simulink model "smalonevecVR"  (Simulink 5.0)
settings: Solver=ode23t  StartTime=0.0  StopTime=4  MaxStep=0.01  RelTol=1e-5  AbsTol=1e-4
InitFcn:
  | smalonevecdef
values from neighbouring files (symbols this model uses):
  Ef = parEf(m)    [Ccurverun.m]
  Ra = .95    (= 0.95)    [altwdgs.m]    (also in Ccurverun.m = 0.018)
  wo = 2*pi*freq0    [calc0.m]    (also in IMabc2.m = 376.991118431; imabcparam.m = 376.991118431; IMabcrun0.m = 376.991118431; IMabcrun1.m = 376.991118431)
undefined symbols (not defined in the file or in its folder): fa0, fk0, L_1, phif0, Rf, Rkd, Rkq, vf0

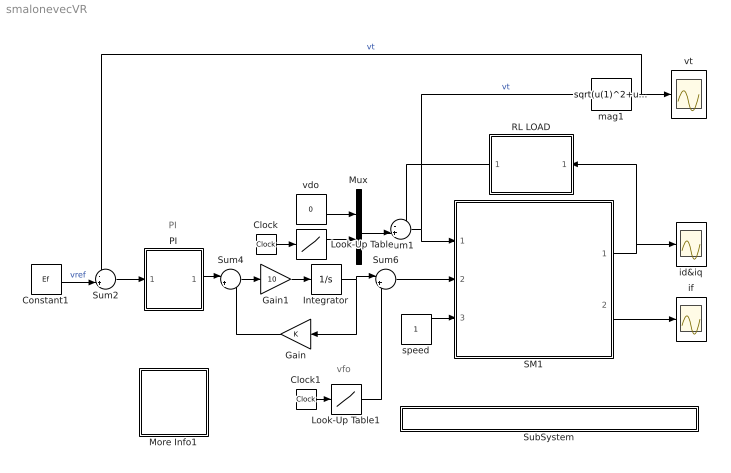
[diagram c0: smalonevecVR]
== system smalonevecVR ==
  note: vfo
  note: PI
  Clock : Clock
  Clock1 : Clock
  Constant1 : Constant  Value=Ef
  Gain : Gain  Orientation=left
  Gain1 : Gain  Gain=10
  Integrator : Integrator
  Look-Up Table : Lookup  InputValues=[0 0.5 0.51 20]  OutputValues=[Ef Ef 0 0]
  Look-Up Table1 : Lookup  InputValues=[0 0.5 0.54 20]  OutputValues=[vf0 vf0 0 0]
  More Info1 : Subsystem
  Mux : Mux  Inputs=2
  PI : Subsystem
  RL LOAD : Subsystem  Orientation=left  mask{Rline=0.4, Lline=1, wo=2*pi*60}
      mask prompts: Rline "Rline [ pu]"; Lline "Lline [pu]"; wo "wo [rad/s]"
  SM1 : Subsystem
  SubSystem : Subsystem
  Sum1 : Sum  Inputs=-+|
  Sum2 : Sum  Inputs=-+|
  Sum4 : Sum  Inputs=|+-
  Sum6 : Sum  Inputs=|++
  id&iq : Scope
  if : Scope
  mag1 : Fcn  Expr=sqrt(u(1)^2+u(2)^2)
  speed : Constant
  vdo : Constant  Value=0
  vt : Scope
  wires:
  SM1/2(if) -> if/1
  speed/1 -> SM1/3(wm)
  Look-Up Table/1 -> Mux/2
  Mux/1 -> Sum1/2
  RL LOAD/1(v_out) -> Sum1/1
  Sum1/1 -> SM1/1(vs), mag1/1  "vt"
  SM1/1(ia) -> RL LOAD/1(i_in), id&iq/1
  Clock/1 -> Look-Up Table/1
  Gain/1 -> Sum4/2
  Constant1/1 -> Sum2/2  "vref"
  Sum2/1 -> PI/1(we)
  PI/1(wr) -> Sum4/1
  Sum4/1 -> Gain1/1
  Gain1/1 -> Integrator/1
  Integrator/1 -> Gain/1, Sum6/1
  Clock1/1 -> Look-Up Table1/1
  Look-Up Table1/1 -> Sum6/2
  Sum6/1 -> SM1/2(vf)
  mag1/1 -> vt/1, Sum2/1  "vt"
  vdo/1 -> Mux/1

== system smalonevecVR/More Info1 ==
  note: The generator runs under open-cicuit conditions when an inductive-resistive load is suddenly applied
  note: Synchronous generator with voltage regulator

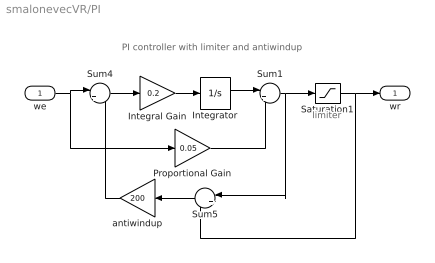
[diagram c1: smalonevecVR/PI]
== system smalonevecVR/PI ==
  note: PI controller with limiter and antiwindup
  note: limiter
  we : Inport
  Integral Gain : Gain  Gain=0.2
  Integrator : Integrator
  Proportional Gain : Gain  Gain=0.05
  Saturation1 : Saturate  UpperLimit=0.003  LowerLimit=-0.003
  Sum1 : Sum  Inputs=|++
  Sum4 : Sum  Inputs=|+-
  Sum5 : Sum  Orientation=left  Inputs=|+-
  antiwindup : Gain  Orientation=left  Gain=200
  wr : Outport
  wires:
  Saturation1/1 -> Sum5/2, wr/1
  antiwindup/1 -> Sum4/2
  Sum5/1 -> antiwindup/1
  Sum1/1 -> Sum5/1, Saturation1/1
  Sum4/1 -> Integral Gain/1
  we/1 -> Proportional Gain/1, Sum4/1
  Proportional Gain/1 -> Sum1/2
  Integrator/1 -> Sum1/1
  Integral Gain/1 -> Integrator/1

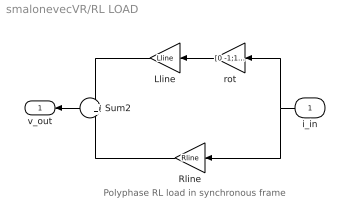
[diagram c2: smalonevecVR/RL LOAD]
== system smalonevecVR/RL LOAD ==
  note: Polyphase RL load in synchronous frame
  i_in : Inport  Orientation=left
  Lline : Gain  Orientation=left  Gain=Lline
  Rline : Gain  Orientation=left  Gain=Rline
  Sum2 : Sum  Orientation=left
  rot : Gain  Orientation=left  Gain=[0 -1;1 0]  Multiplication=Matrix(K*u)
  v_out : Outport  Orientation=left
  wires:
  Sum2/1 -> v_out/1
  i_in/1 -> rot/1, Rline/1
  rot/1 -> Lline/1
  Lline/1 -> Sum2/1
  Rline/1 -> Sum2/2

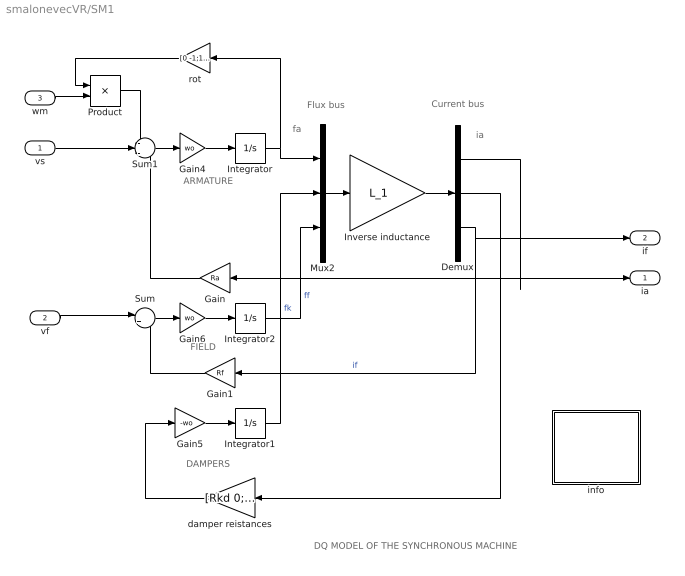
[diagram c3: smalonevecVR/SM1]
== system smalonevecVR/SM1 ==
  note: DAMPERS
  note: ARMATURE
  note: fa
  note: ia
  note: FIELD
  note: DQ MODEL OF THE SYNCHRONOUS MACHINE
  note: Flux bus
  note: Current bus
  vs : Inport
  vf : Inport  Port=2
  wm : Inport  Port=3
  Demux : Demux  Outputs=3
  Gain : Gain  Orientation=left  Gain=Ra
  Gain1 : Gain  Orientation=left  Gain=Rf
  Gain4 : Gain  Gain=wo
  Gain5 : Gain  Gain=-wo
  Gain6 : Gain  Gain=wo
  Integrator : Integrator  InitialCondition=fa0
  Integrator1 : Integrator  InitialCondition=fk0
  Integrator2 : Integrator  InitialCondition=phif0
  Inverse inductance : Gain  Gain=L_1  Multiplication=Matrix(K*u)
  Mux2 : Mux  Inputs=3
  Product : Product
  Sum : Sum  Inputs=|+-
  Sum1 : Sum  Inputs=-+-
  damper reistances : Gain  Orientation=left  Gain=[Rkd 0;0 Rkq]  Multiplication=Matrix(K*u)
  info : Subsystem
  rot : Gain  Orientation=left  Gain=[0 -1;1 0]  Multiplication=Matrix(K*u)
  ia : Outport
  if : Outport  Port=2
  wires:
  Product/1 -> Sum1/1
  rot/1 -> Product/1
  wm/1 -> Product/2
  Gain5/1 -> Integrator1/1
  damper reistances/1 -> Gain5/1
  Integrator/1 -> Mux2/1, rot/1
  Sum1/1 -> Gain4/1
  Gain4/1 -> Integrator/1
  vs/1 -> Sum1/2
  Gain/1 -> Sum1/3
  Gain6/1 -> Integrator2/1
  Sum/1 -> Gain6/1
  vf/1 -> Sum/1
  Gain1/1 -> Sum/2
  Demux/1 -> Gain/1, ia/1
  Mux2/1 -> Inverse inductance/1
  Inverse inductance/1 -> Demux/1
  Integrator1/1 -> Mux2/2  "fk"
  Integrator2/1 -> Mux2/3  "ff"
  Demux/2 -> damper reistances/1
  Demux/3 -> if/1, Gain1/1  "if"

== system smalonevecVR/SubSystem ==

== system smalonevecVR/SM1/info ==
  note: This demonstration illustrates the dynamics of a synchronous generator, initially at no load, following a three-phase short circuit at the terminals.
  note: Synchronous machine transients under shortcircuit
